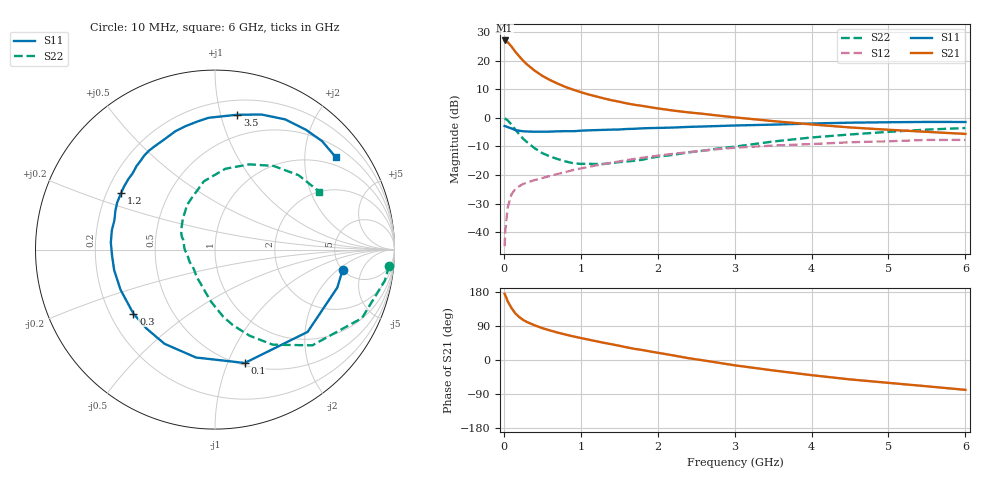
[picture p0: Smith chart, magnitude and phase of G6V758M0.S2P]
! SIEMENS Small Signal Semiconductors
! BFG193
! Si NPN RF Bipolar Junction Transistor in SOT223
! VCE = 0.75 V  IC = 8 mA
! Common Emitter S-Parameters:  August  1996
# GHz  S  MA  R  50
!  f  S11  S21  S12  S22
! GHz  MAG  ANG  MAG  ANG  MAG  ANG  MAG  ANG
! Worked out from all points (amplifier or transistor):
!   36 points, 10 MHz to 6 GHz, reference 50 ohm
!   highest |S21| = 27.1 dB at 10 MHz (marker M1)
!   |S21| within 3 dB of that: start of sweep to 123.5 MHz
!   unconditionally stable (mu >= 1): 875.1 MHz to 3.776 GHz
!   at 250 MHz: K = 0.48, MSG = 21.6 dB, |S12| = -23.1 dB
!   at 1.4 GHz: K = 1.09, MAG = 9.1 dB, |S12| = -15.7 dB
!   at 6 GHz: K = 0.98, MSG = 1.0 dB, |S12| = -7.7 dB
!   S11 on the Smith chart (normalised r, x): 10 MHz: 5.03, -2.33; 100 MHz: 0.52, -1.15; 300 MHz: 0.30, -0.32; 1.2 GHz: 0.26, +0.26; 3.5 GHz: 0.32, +1.13; 6 GHz: 0.76, +2.76
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0.01  0.7202 -8.9  22.58 174.6  0.0057 87.5  0.9746 -5.3
0.02  0.7137 -17.2  22.36 170.4  0.011 81.5  0.9616 -10.4
0.05  0.6904 -41.6  21.02 154.9  0.027 69.9  0.9033 -25.0
0.1  0.6531 -75.3  17.64 137.1  0.0461 58.5  0.7608 -44.5
0.15  0.6105 -100.0  14.31 122.7  0.0573 48.4  0.6202 -58.7
0.2  0.5955 -118.2  11.94 113.4  0.0638 44.5  0.5163 -68.2
0.25  0.5822 -131.2  10.03 105.9  0.0696 41.6  0.4324 -76.7
0.3  0.5778 -141.9  8.627 100.3  0.0737 40.7  0.3778 -82.9
0.4  0.5719 -157.0  6.712 91.6  0.0815 39.5  0.2941 -93.8
0.5  0.5733 -168.5  5.434 84.1  0.0885 39.4  0.2419 -102.9
0.6  0.5744 -176.6  4.589 78.0  0.0964 40.0  0.211 -111.1
0.7  0.5819 176.0  3.97 72.3  0.1044 40.1  0.1902 -119.7
0.8  0.5847 169.3  3.477 67.2  0.1126 39.9  0.1733 -128.7
1.1  0.6049 154.2  2.568 53.8  0.1385 38.8  0.1572 -152.7
1.2  0.6106 149.1  2.37 49.6  0.1475 38.1  0.156 -160.4
1.6  0.6386 133.2  1.788 33.3  0.1829 32.7  0.1727 174.4
2.2  0.6767 114.3  1.342 12.2  0.2352 22.2  0.225 145.7
2.8  0.7206 97.7  1.091 -7.6  0.2857 9.9  0.2928 122.3
3.5  0.7617 80.6  0.877 -27.5  0.3275 -6.4  0.3856 99.2
4.5  0.824 61.7  0.68 -51.2  0.3745 -25.3  0.5123 68.0
5.5  0.8492 45.4  0.569 -69.4  0.4112 -47.7  0.6233 41.7
6  0.8469 37.5  0.524 -78.8  0.4115 -60.4  0.6644 29.1
